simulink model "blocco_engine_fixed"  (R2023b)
settings: Solver=VariableStepAuto  StartTime=0.0  StopTime=10.0  RelTol=1e-3
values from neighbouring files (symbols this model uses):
  gear_ratio = 10    [motor_map.m]
  mot_alpha_bp = alpha_vec * 100    [motor_map.m]
  mot_n_bp = n_vec    [motor_map.m]
  mot_T_table = T_map.'    [motor_map.m]
libraries: slpidlib x1

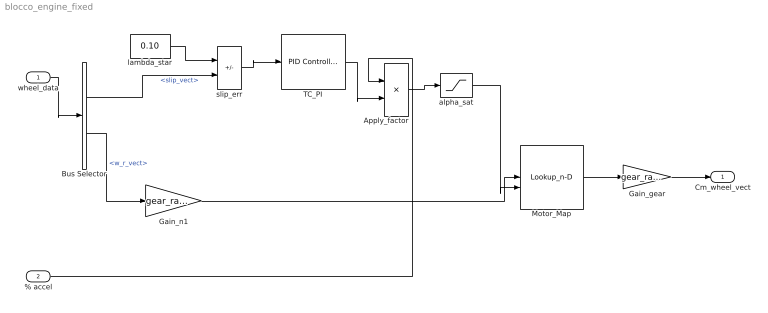
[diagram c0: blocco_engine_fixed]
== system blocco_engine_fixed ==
  wheel_data : Inport
  % accel : Inport  Port=2
  Apply_factor : Product  Inputs=**
  Bus Selector : BusSelector  OutputSignals=slip_vect,w_r_vect
  Gain_gear : Gain  Gain=gear_ratio
  Gain_n1 : Gain  Gain=gear_ratio*60/(2*pi)
  Motor_Map : Lookup_n-D  BreakpointsForDimension1=mot_n_bp  BreakpointsForDimension2=mot_alpha_bp  BreakpointsForDimension3=[5, 7]  Table=mot_T_table  ExtrapMethod=Clip  InternalRulePriority=Speed  RndMeth=Simplest
  TC_PI : slpidlib/PID Controller  Controller=PI  Form=Parallel  TimeDomain=Continuous-time  UseExternalTs=off  SampleTime=-1  IntegratorMethod=Forward Euler  FilterMethod=Forward Euler  ControllerParametersSource=internal  P=4  I=15  UseKiTs=off  D=0  N=100  UseFilter=on  TunerSelectOption=Transfer Function Based (PID Tuner App)  InitialConditionSource=internal  InitialConditionForIntegrator=1  InitialConditionForFilter=0  DifferentiatorICPrevScaledInput=0  ExternalReset=none  TrackingMode=off  Kt=1  LimitOutput=on  SatLimitsSource=internal  UpperSaturationLimit=1  LowerSaturationLimit=0  LinearizeAsGain=on  AntiWindupMode=clamping  Kb=1  LimitIntegrator=off  UpperIntegratorSaturationLimit=inf  LowerIntegratorSaturationLimit=-inf  POutMin=[]  POutMax=[]  IOutMin=[]  IOutMax=[]  DOutMin=[]  DOutMax=[]  NOutMin=[]  NOutMax=[]  SumOutMin=[]  SumOutMax=[]  SaturationOutMin=[]  SaturationOutMax=[]  PParamMin=[]  PParamMax=[]  IParamMin=[]  IParamMax=[]  DParamMin=[]  DParamMax=[]  NParamMin=[]  NParamMax=[]  KbParamMin=[]  KbParamMax=[]  KtParamMin=[]  KtParamMax=[]  KbOutMin=[]  KbOutMax=[]  KtOutMin=[]  KtOutMax=[]  IntegratorOutMin=[]  IntegratorOutMax=[]  FilterOutMin=[]  FilterOutMax=[]  SumI1OutMin=[]  SumI1OutMax=[]  SumI2OutMin=[]  SumI2OutMax=[]  SumI3OutMin=[]  SumI3OutMax=[]  SumI4OutMin=[]  SumI4OutMax=[]  SumDOutMin=[]  SumDOutMax=[]  DifferentiatorOutMin=[]  DifferentiatorOutMax=[]  FilterDiffOutCoefMin=[]  FilterDiffOutCoefMax=[]  ReciprocalOutMin=[]  ReciprocalOutMax=[]  SumDenOutMin=[]  SumDenOutMax=[]  SumNumOutMin=[]  SumNumOutMax=[]  DivideOutMin=[]  DivideOutMax=[]  UdiffTsProdOutMin=[]  UdiffTsProdOutMax=[]  NTsProdOutMin=[]  NTsProdOutMax=[]  UintegralTsProdOutMin=[]  UintegralTsProdOutMax=[]  UngainTsProdOutMin=[]  UngainTsProdOutMax=[]  ClampingZeroOutDataTypeStr=Inherit: Inherit via back propagation  ClampingZeroOutMin=[]  ClampingZeroOutMax=[]  FilterDenConstantOutDataTypeStr=Inherit: Inherit via back propagation  FilterDenConstantOutMin=[]  FilterDenConstantOutMax=[]  PCopyOutDataTypeStr=Inherit: Inherit via back propagation  PCopyOutMin=[]  PCopyOutMax=[]  NCopyOutDataTypeStr=Inherit: Inherit via back propagation  NCopyOutMin=[]  NCopyOutMax=[]  IntegratorContinuousStateAttributes=''  IntegratorStateMustResolveToSignalObject=off  IntegratorRTWStateStorageClass=Auto  FilterContinuousStateAttributes=''  FilterStateMustResolveToSignalObject=off  FilterRTWStateStorageClass=Auto  ParallelPVariant=InternalParameters  IdealPVariant=Disabled  IVariant=InternalParameters  DVariant=Disabled  IntegratorVariant=Continuous  SatVariant=Enabled  AWVariant=ContClampingParallel  PCopyVariant=Disabled  TRVariant=Disabled  FdbkBlocksVariant=Forward  IdealPFdbkVariant=Disabled  SatFdbkVariant=Disabled  DerivativeFilterVariant=Disabled  NVariant=Disabled  NCopyVariant=Disabled_SignalSpec  FilterICVariant=Disabled  IntegratorICVariant=InternalICs  ExternalResetVariant=Disabled  TRSumVariant=Passthrough  SumFdbkVariant=Disabled  SumVariant=Sum_PI  TsampFilterVariant=InternalTs  TsampNgainVariant=Passthrough  TsampIntegralVariant=Disabled_SignalSpec  ExternalSaturationOutDataTypeStr=Inherit: Same as second input
  alpha_sat : Saturate  UpperLimit=100  LowerLimit=0
  lambda_star : Constant  Value=0.10
  slip_err : Sum  Inputs=+-
  Cm_wheel_vect : Outport
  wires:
  wheel_data/1 -> Bus Selector/1
  Bus Selector/1 -> slip_err/2  "<slip_vect>"
  Bus Selector/2 -> Gain_n1/1  "<w_r_vect>"
  lambda_star/1 -> slip_err/1
  slip_err/1 -> TC_PI/1
  TC_PI/1 -> Apply_factor/2
  % accel/1 -> Apply_factor/1
  Apply_factor/1 -> alpha_sat/1
  Gain_n1/1 -> Motor_Map/1
  alpha_sat/1 -> Motor_Map/2
  Motor_Map/1 -> Gain_gear/1
  Gain_gear/1 -> Cm_wheel_vect/1
